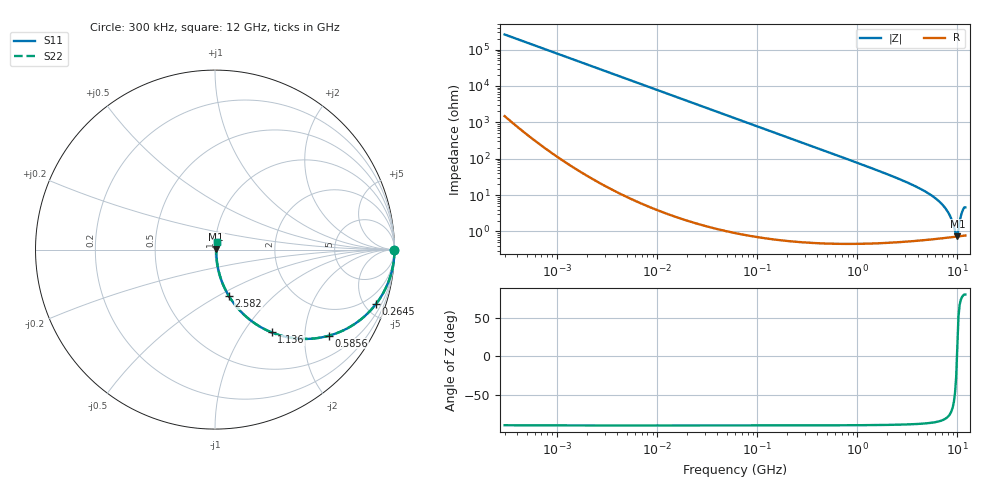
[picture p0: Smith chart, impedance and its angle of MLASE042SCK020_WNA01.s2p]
! MLASE042SCK020_WNA01  S-PARAMETER MODEL  ( General Type )
! Model Generated by TAIYO YUDEN Corporation (http://www.ty-top.com)
! Version 2.0
! TAIYO YUDEN Control No. 120810
! Copyright(c) 2011 TAIYO YUDEN CO.,LTD. All Rights Reserved.
! Product Description (link to TY-COMPAS)
! https://ds.yuden.co.jp/TYCOMPAS/or/detail?pn=MLASE042SCK020AWNA01&u=M
! Products Name : Multilayer Ceramic Capacitors
! Characteristics :
!  Capacitance : 2 pF , Rated Voltage : 16V , TCC : CK / C0K
!  Case Size : 0.4 x 0.2 / 0.016 x 0.008 [mm/inch] , Thickness : 0.2 / 0.008 [mm/inch]
!  (Conditions: Temperature = 25 degC , DC Bias Current/Voltage = 0A / 0V)
! External Node Assignments :
!  1  o---| |---o  2
! GND o---------o GND
! Frequency Range : 0.3MHz  -  12000MHz  [ 401 STEP ]
# MHz S RI R 50
! Freq[MHz].  S11 Real  S11 Imag  S21 Real  S21 Imag  S12 Real  S12 Imag  S22 Real  S22 Imag
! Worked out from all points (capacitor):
!   401 points, 300 kHz to 12 GHz, reference 50 ohm
!   read as one part in series: C = 2.05 pF near 316.3 kHz
!   lowest |Z| = 745 mohm at 9.969 GHz (marker M1)
!   series resonance near 9.889 GHz, so ESL is about 130 pH
!   S11 on the Smith chart (normalised r, x): 300 kHz: open; 264.5 MHz: 1.01, -5.88; 585.6 MHz: 1.01, -2.65; 1.136 GHz: 1.01, -1.35; 2.582 GHz: 1.01, -0.56; 12 GHz: 1.02, +0.09
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0.3  1 -0.000386  2.35e-06 0.000386  2.35e-06 0.000386  1 -0.000386
1.769972  1 -0.00228  7.32e-06 0.00228  7.32e-06 0.00228  1 -0.00228
10.44266  0.9998 -0.0134  0.000187 0.0134  0.000187 0.0134  0.9998 -0.0134
60  0.994 -0.0767  0.00597 0.0767  0.00597 0.0767  0.994 -0.0767
129.3602  0.9729 -0.1618  0.0271 0.1618  0.0271 0.1618  0.9729 -0.1618
264.5085  0.8958 -0.3046  0.1042 0.3046  0.1042 0.3046  0.8958 -0.3046
353.9943  0.8275 -0.3767  0.1725 0.3767  0.1725 0.3767  0.8275 -0.3767
585.5907  0.6362 -0.4793  0.3638 0.4793  0.3638 0.4793  0.6362 -0.4793
804.7407  0.4799 -0.4972  0.5201 0.4972  0.5201 0.4972  0.4799 -0.4972
1135.593  0.3149 -0.4611  0.6851 0.4611  0.6851 0.4611  0.3149 -0.4611
2088.533  0.1159 -0.3132  0.8841 0.3132  0.8841 0.3132  0.1159 -0.3132
2581.562  0.0772 -0.258  0.9228 0.258  0.9228 0.258  0.0772 -0.258
4385.161  0.0253 -0.1384  0.9747 0.1384  0.9747 0.1384  0.0253 -0.1384
6354.153  0.0114 -0.0711  0.9886 0.0711  0.9886 0.0711  0.0114 -0.0711
7854.144  0.00804 -0.0366  0.992 0.0366  0.992 0.0366  0.00804 -0.0366
8503.825  0.00744 -0.0242  0.9926 0.0242  0.9926 0.0242  0.00744 -0.0242
9454.42  0.00715 -0.00771  0.9928 0.00771  0.9928 0.00771  0.00715 -0.00771
9708.23  0.00717 -0.0036  0.9928 0.0036  0.9928 0.0036  0.00717 -0.0036
9968.853  0.00723 0.00158  0.9928 -0.00158  0.9928 -0.00158  0.00723 0.00158
10236.47  0.00737 0.00923  0.9926 -0.00923  0.9926 -0.00923  0.00737 0.00923
11083.22  0.00853 0.0321  0.9915 -0.0321  0.9915 -0.0321  0.00853 0.0321
12000  0.0097 0.0445  0.9903 -0.0445  0.9903 -0.0445  0.0097 0.0445
